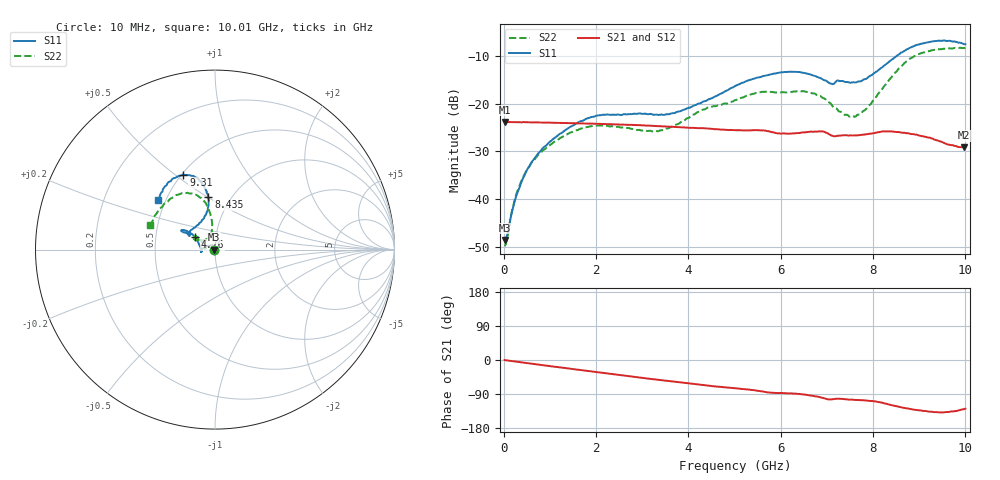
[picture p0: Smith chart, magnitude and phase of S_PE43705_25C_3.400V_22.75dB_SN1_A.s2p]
! Device ID: PE43705
! Serial: 1
! Insertion: A
! Impedance: 50 ohm
! Temp: 25C
! VDD: 3.400V
! Attenuation Step: 22.75dB
#  Hz  S  RI  R  50
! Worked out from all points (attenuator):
!   401 points, 10 MHz to 10.01 GHz, reference 50 ohm
!   highest |S21| = -23.80 dB at 10 MHz (marker M1); lowest = -29.1 dB at 9.985 GHz (marker M2)
!   lowest |S11| = -48.5 dB at 10 MHz (marker M3), VSWR 1.01, Z = 49.6 + j0.0382 ohm
!   |S11| at or under -10 dB: start of sweep to 8.518 GHz
!   |S22| runs from -49.8 to -8.3 dB; largest |S21 - S12| = 0.00086
!   S11 on the Smith chart (normalised r, x): 10 MHz: 0.99, +0.00; 4.76 GHz: 0.79, +0.11; 8.435 GHz: 0.79, +0.50; 9.31 GHz: 0.51, +0.53; 10.01 GHz: 0.46, +0.31
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1e7  -0.00373 0.000385  0.0645 -0.000201  0.0646 -0.000243  -0.00319 0.000478
8.5e7  -0.0035 0.00296  0.0643 -0.00167  0.0643 -0.00166  -0.00261 0.00339
2.6e8  -0.00517 0.00941  0.064 -0.00489  0.0639 -0.00485  -0.00396 0.0105
5.35e8  -0.0125 0.0178  0.0631 -0.0098  0.0632 -0.00981  -0.00992 0.0192
1.01e9  -0.0346 0.0214  0.0607 -0.0179  0.0607 -0.0179  -0.0281 0.0246
1.685e9  -0.0655 0.0083  0.0555 -0.0281  0.0555 -0.0281  -0.0526 0.0169
2.185e9  -0.0764 -0.00724  0.0504 -0.0349  0.0504 -0.0349  -0.0581 0.00727
3.36e9  -0.0761 -0.00621  0.0353 -0.0463  0.0353 -0.0462  -0.0502 0.0131
4.76e9  -0.1111 0.071  0.0168 -0.0509  0.0169 -0.0508  -0.0812 0.0583
5.01e9  -0.127 0.0857  0.0141 -0.0509  0.0142 -0.051  -0.0887 0.0635
5.535e9  -0.1583 0.1031  0.00749 -0.0521  0.00767 -0.0522  -0.1083 0.0742
6.01e9  -0.1827 0.1091  0.0025 -0.0486  0.00251 -0.0488  -0.1107 0.071
6.685e9  -0.1747 0.0956  -0.00382 -0.0509  -0.00394 -0.0508  -0.1146 0.0584
7.11e9  -0.1402 0.0804  -0.011 -0.0451  -0.0109 -0.0449  -0.0815 0.0529
7.61e9  -0.0974 0.136  -0.0122 -0.0449  -0.0122 -0.0448  -0.0375 0.0626
7.885e9  -0.0605 0.1764  -0.0142 -0.0459  -0.0142 -0.0461  -0.0225 0.0897
8.36e9  -0.0345 0.2752  -0.0239 -0.0454  -0.0239 -0.0455  -0.0208 0.1782
8.435e9  -0.037 0.2927  -0.0253 -0.0442  -0.0253 -0.0445  -0.0249 0.1962
8.86e9  -0.0883 0.3861  -0.0312 -0.0366  -0.0306 -0.037  -0.0882 0.2932
9.31e9  -0.1758 0.4158  -0.0315 -0.0291  -0.0315 -0.0293  -0.1897 0.312
9.985e9  -0.3091 0.285  -0.0222 -0.0271  -0.0227 -0.0271  -0.353 0.1485
1.001e10  -0.316 0.2775  -0.022 -0.0278  -0.0222 -0.0278  -0.3609 0.1371
